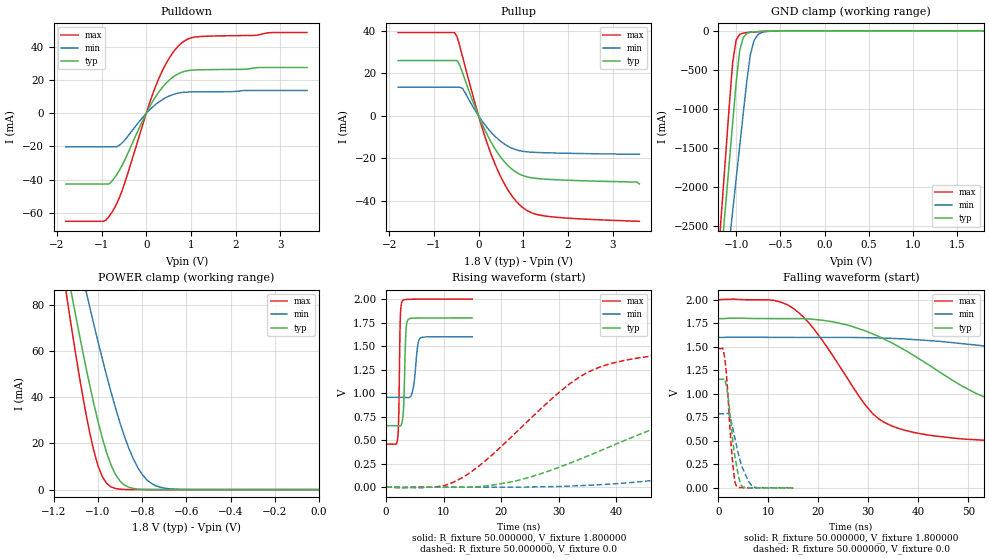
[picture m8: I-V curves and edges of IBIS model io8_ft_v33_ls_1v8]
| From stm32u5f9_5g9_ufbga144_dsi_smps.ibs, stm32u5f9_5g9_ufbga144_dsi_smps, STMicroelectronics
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|   Model io8_ft_v33_ls_1v8
[Model]  io8_ft_v33_ls_1v8
Model_type I/O
Polarity   Non-Inverting
Enable   Active-Low
Vinl =   0.540000V
Vinh =   1.260000V
Vmeas =  0.900000V
Cref =   50.000000pF
Rref =   100.000000M
Vref =   0.0V
C_comp   3.087500pF   3.086600pF   3.135700pF
[Temperature Range]   25.000000   0.140000k   -40.000000
[Pullup Reference]   1.800000V   1.600000V   2.000000V
[Pulldown Reference]   0.0V   0.0V   0.0V
[POWER Clamp Reference]   1.800000V   1.600000V   2.000000V
[GND Clamp Reference]   0.0V   0.0V   0.0V
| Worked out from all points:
|   slope of the pulldown table from 0 to 0.27 V, typ, clamps not added: 21.7 ohm
|   slope of the pullup table from 0 to 0.27 V, typ, clamps not added: 22.6 ohm
|   GND clamp passes 1 mA (typ) near -0.51 V on its own axis
|   POWER clamp passes 1 mA (typ) near -0.86 V on its own axis
|   rising waveform, R_fixture 50.000000, V_fixture 1.800000: 20-80 % time 315ps typ, 622ps min, 226ps max; typ from 0.654 V to 1.8 V
|   rising waveform, R_fixture 50.000000, V_fixture 0.0: 20-80 % time 31.3ns typ, 66.8ns min, 16.5ns max; typ from 0 V to 1.16 V
|   falling waveform, R_fixture 50.000000, V_fixture 1.800000: 20-80 % time 24.5ns typ, 55.4ns min, 12.3ns max; typ from 1.8 V to 0.654 V
|   falling waveform, R_fixture 50.000000, V_fixture 0.0: 20-80 % time 1.6ns typ, 2.38ns min, 1.17ns max; typ from 1.16 V to 0 V
[Pulldown]
|Voltage   I(typ)   I(min)   I(max)
-1.8V     -42.74mA   -20.21mA   -65.25mA
-960mV    -42.74mA   -20.21mA   -65.25mA
-780mV    -41.3mA    -20.21mA   -60.25mA
-660mV    -37mA      -20.2mA    -54.5mA
-540mV    -31.39mA   -17.82mA   -46.65mA
0V        -10fA      0A         10fA
240mV     11.28mA    6.002mA    18.38mA
480mV     19.18mA    10.02mA    31.83mA
780mV     24.67mA    12.5mA     42.21mA
960mV     25.9mA     12.9mA     45.21mA
1.14V     26.24mA    12.99mA    46.23mA
3.6V      27.69mA    13.82mA    48.79mA
[Pullup]
|Voltage   I(typ)   I(min)   I(max)
-1.8V     26.06mA    13.5mA     39.24mA
-540mV    26.06mA    13.5mA     39.24mA
-480mV    26.06mA    13.5mA     37.19mA
-360mV    20.34mA    12.93mA    27.94mA
0V        590fA      222pA      0A
300mV     -13.1mA    -8.158mA   -19.11mA
480mV     -18.98mA   -11.71mA   -27.97mA
660mV     -23.42mA   -14.29mA   -34.95mA
1.02V     -28.29mA   -16.75mA   -43.65mA
1.26V     -29.33mA   -17.15mA   -46.11mA
1.62V     -29.92mA   -17.41mA   -47.45mA
3.6V      -32mA      -18mA      -49.6mA
[GND_clamp]
|Voltage   I(typ)   I(min)   I(max)
-1.8V     -9.707A    -9.942A    -9.774A
-1.2V     -3.309A    -4.006A    -2.864A
-1.16V    -2.777A    -3.584A    -2.239A
-1.12V    -2.246A    -3.162A    -1.614A
-1.04V    -1.186A    -2.319A    -408.6mA
-1V       -663.9mA   -1.898A    -117.8mA
-960mV    -254mA     -1.478A    -45.14mA
-920mV    -86.03mA   -1.06A     -28.58mA
-840mV    -19.12mA   -308.9mA   -18.74mA
-800mV    -13.39mA   -130.8mA   -15.31mA
-720mV    -7.948mA   -25.37mA   -9.381mA
1.8V      0A         14.97nA    0A
[POWER_clamp]
|Voltage   I(typ)   I(min)   I(max)
-1.8V     470.8mA    433.7mA    554.6mA
-1.14V    95.25mA    122.7mA    82.82mA
-1.12V    84.97mA    114mA      70.27mA
-1.06V    55.51mA    88.42mA    35.67mA
-1.04V    46.34mA    80.15mA    25.76mA
-1V       29.51mA    64.13mA    10.3mA
-940mV    10.39mA    41.86mA    1.109mA
-900mV    3.624mA    28.77mA    182.8uA
-840mV    490.7uA    13.24mA    11.35uA
-800mV    116.8uA    6.532mA    1.77uA
-740mV    13.2uA     1.723mA    109.3nA
0V        0A         18.72nA    0A
[Ramp]
| variable   typ   min   max
dV/dt_r  0.69306/31.25872n   0.47201/66.68140n   0.88872/16.44123n
dV/dt_f  0.68762/24.46612n   0.38678/55.36222n   0.92481/12.26159n
R_load = 50.000000
[Rising Waveform]
R_fixture= 50.000000
V_fixture= 1.800000
V_fixture_min= 1.600000
V_fixture_max= 2.000000
|time   V(typ)   V(min)   V(max)
0s        654mV      955.4mV    458.7mV
2.012ns   653.5mV    955.4mV    524.4mV
2.192ns   652.2mV    955.4mV    777.1mV
2.462ns   651.6mV    955.4mV    1.801V
2.793ns   700.6mV    955.4mV    1.979V
3.063ns   885mV      955.2mV    1.993V
3.423ns   1.634V     954.1mV    1.996V
3.814ns   1.781V     951.7mV    1.997V
5.946ns   1.799V     1.587V     2V
14.95ns   1.8V       1.6V       2V
[Rising Waveform]
R_fixture= 50.000000
V_fixture= 0.0
V_fixture_min= 0.0
V_fixture_max= 0.0
|time   V(typ)   V(min)   V(max)
0s        2.236nV    145.8nV    1.532nV
13.01ns   773.6uV    -136.9uV   93.59mV
23.02ns   73.59mV    888.9uV    607.4mV
31.03ns   233.8mV    9.424mV    1.057V
37.04ns   382.1mV    26.19mV    1.275V
59.06ns   877.2mV    166.2mV    1.451V
91.09ns   1.107V     434.3mV    1.478V
129.1ns   1.147V     647.7mV    1.481V
167.2ns   1.154V     737.1mV    1.481V
498.5ns   1.155V     786.8mV    1.481V
[Falling Waveform]
R_fixture= 50.000000
V_fixture= 1.800000
V_fixture_min= 1.600000
V_fixture_max= 2.000000
|time   V(typ)   V(min)   V(max)
0s        1.8V       1.6V       2V
11.01ns   1.8V       1.6V       1.994V
15.02ns   1.8V       1.6V       1.907V
20.02ns   1.787V     1.6V       1.624V
30.03ns   1.656V     1.597V     838.9mV
34.03ns   1.559V     1.591V     673.5mV
56.06ns   913.1mV    1.488V     496.8mV
97.1ns    693.4mV    1.15V      462.2mV
150.2ns   659.9mV    1.012V     458.9mV
498.5ns   654mV      955.4mV    458.7mV
[Falling Waveform]
R_fixture= 50.000000
V_fixture= 0.0
V_fixture_min= 0.0
V_fixture_max= 0.0
|time   V(typ)   V(min)   V(max)
0s        1.155V     786.8mV    1.481V
810.8ps   1.155V     786.8mV    1.485V
1.291ns   1.149V     786.6mV    1.364V
2.012ns   931.9mV    789.8mV    875.2mV
2.763ns   548.1mV    657mV      314.6mV
3.153ns   379.3mV    561.6mV    116.2mV
3.514ns   265.9mV    472mV      28.27mV
4.685ns   18.02mV    229.4mV    2.13mV
6.637ns   1.097mV    24.79mV    316.6uV
14.95ns   2.236nV    145.8nV    1.532nV
